(* Logix 5000 AddOnInstructionDefinition export ACS_CLEAR_START_MOTION; software revision 20.01 *)

ADD_ON_INSTRUCTION ACS_CLEAR_START_MOTION   (* revision 2.0, vendor Tolomatic, Inc *)
// Clears the Start Motion Bit
// Clears Start Motion Timer Enable Line
// Resets Start Motion Timer Accumulator
VAR_IN_OUT
   DriveCMD : SINT; {required}   // ACS.O.CMD
   SMTimerEnable : BOOL; {required}   // Start Motion Timer Enable Line
   SMTimer : TIMER; {required}   // Start Motion Timer
END_VAR
VAR
   OutMask : DINT; {access None}   // Mask used to clear start motion bit
END_VAR

ROUTINE Logic   (* ladder *)
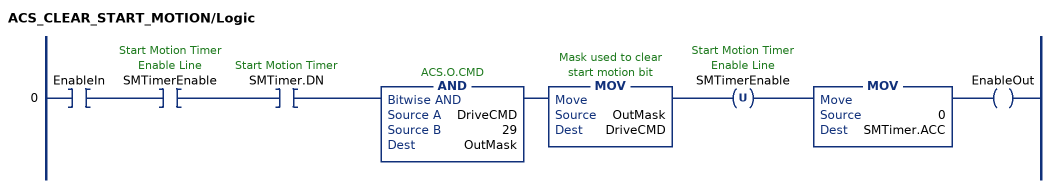
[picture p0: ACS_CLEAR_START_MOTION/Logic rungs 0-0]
   0: XIC(EnableIn)XIC(SMTimerEnable)XIC(SMTimer.DN)AND(DriveCMD,29,OutMask)MOV(OutMask,DriveCMD)OTU(SMTimerEnable)MOV(0,SMTimer.ACC)OTE(EnableOut);
END_ROUTINE
END_ADD_ON_INSTRUCTION
